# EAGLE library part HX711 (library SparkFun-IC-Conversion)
AVIA Semiconductor HX711 - ADC 24-Bit Analog-to-Digital Converter for Weigh Scales Datasheet SparkFun Products: SparkFun Load Cell Amplifier - HX711
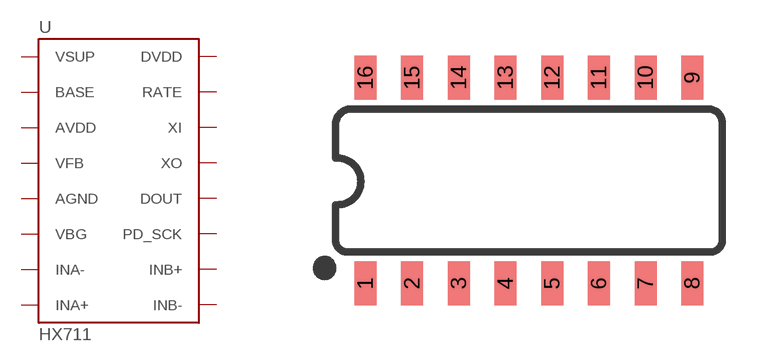
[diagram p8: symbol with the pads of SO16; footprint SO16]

Designator prefix U

## HX711 (PROD_ID: IC-12445; VALUE: HX711)  [SO16]
1  VSUP
2  BASE
3  AVDD
4  VFB
5  AGND
6  VBG
7  INA-
8  INA+
9  INB-
10  INB+
11  PD_SCK
12  DOUT
13  XO
14  XI
15  RATE
16  DVDD

## Footprint SO16 (pad centres in mm)
SOIC -16 Specifications: Pin count: 16 Area: 0.15 width Example device(s): HX711
smd 0.6 x 1.2: 1 -4.445,-2.8; 2 -3.175,-2.8; 3 -1.905,-2.8; 4 -0.635,-2.8; 5 0.635,-2.8; 6 1.905,-2.8; 7 3.175,-2.8; 8 4.445,-2.8; 9 4.445,2.8; 10 3.175,2.8; 11 1.905,2.8; 12 0.635,2.8; 13 -0.635,2.8; 14 -1.905,2.8; 15 -3.175,2.8; 16 -4.445,2.8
